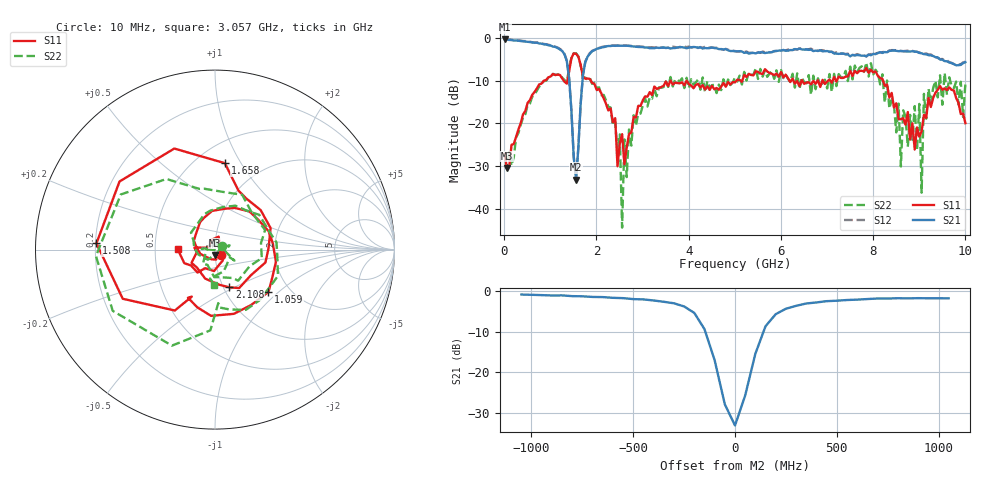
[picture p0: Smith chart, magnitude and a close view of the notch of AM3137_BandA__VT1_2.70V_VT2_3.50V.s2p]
! Date/Time: Tue, Nov 13, 2018 4:48 PM
! Network Analyzer: Agilent Technologies E8364B Rev: A.07.50.67
! Sweep from 0.010 to 10.000 GHz, 201 Points, Sweep Type: LIN
! Power Supply: 2.701 V, -0.002 A
# Hz S DB R 50
!freq MagS11 AngS11 MagS21 AngS21 MagS12 AngS12 MagS22 AngS22
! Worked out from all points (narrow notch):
!   201 points, 10 MHz to 10 GHz, reference 50 ohm
!   highest |S21| = -0.33 dB at 10 MHz (marker M1); lowest = -33.1 dB at 1.558 GHz (marker M2)
!   notch at M2: 30.2 dB deep, 183 MHz wide at half that depth
!   lowest |S11| = -30.4 dB at 59.95 MHz (marker M3), VSWR 1.06, Z = 49.7 - j2.98 ohm
!   |S11| at or under -10 dB: 1.881 GHz to 3.604 GHz (1.723 GHz wide, 62.8 % of centre); 3.958 GHz to 5.037 GHz (1.079 GHz wide, 24 % of centre); 8.215 GHz to end of sweep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
!   |S22| runs from -44.4 to -3.6 dB; largest |S21 - S12| = 0.032
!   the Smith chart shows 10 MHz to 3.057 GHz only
!   S11 on the Smith chart (normalised r, x): 10 MHz: 1.07, -0.06; 1.059 GHz: 1.56, -0.86; 1.508 GHz: 0.20, +0.03; 1.658 GHz: 0.68, +0.86; 2.108 GHz: 1.06, -0.47; 3.057 GHz: 0.66, +0.00
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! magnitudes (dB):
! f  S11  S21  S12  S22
! 10 MHz  -27.2  -0.3  -0.3  -26.9
! 59.95 MHz  -30.4  -0.4  -0.2  -30.7
! 1.059 GHz  -8.4  -2.0  -2.0  -8.4
! 1.359 GHz  -10.7  -5.4  -5.2  -10.5
! 1.508 GHz  -3.6  -27.9  -27.7  -3.6
! 1.558 GHz  -3.7  -33.1  -32.8  -3.6
! 1.658 GHz  -6.3  -15.5  -15.4  -6.4
! 1.708 GHz  -9.0  -8.7  -8.6  -9.2
! 2.108 GHz  -13.0  -2.2  -2.1  -13.4
! 2.508 GHz  -24.7  -1.8  -1.7  -22.6
! 2.557 GHz  -22.5  -1.8  -1.7  -44.4
! 2.607 GHz  -29.6  -1.8  -1.7  -23.7
! 3.057 GHz  -13.6  -2.2  -2.2  -14.1
! 3.357 GHz  -11.7  -2.3  -2.2  -11.6
! 5.005 GHz  -10.4  -3.1  -3.0  -9.2
! 6.703 GHz  -10.0  -3.1  -2.9  -8.8
! 8.352 GHz  -13.9  -3.0  -2.9  -16.5
! 8.601 GHz  -19.0  -3.0  -3.0  -30.1
! 9.001 GHz  -23.1  -3.5  -3.4  -15.4
! 9.051 GHz  -21.8  -3.6  -3.4  -36.2
! 9.101 GHz  -18.0  -3.8  -3.6  -13.1
! 10 GHz  -19.9  -5.6  -5.5  -10.7
